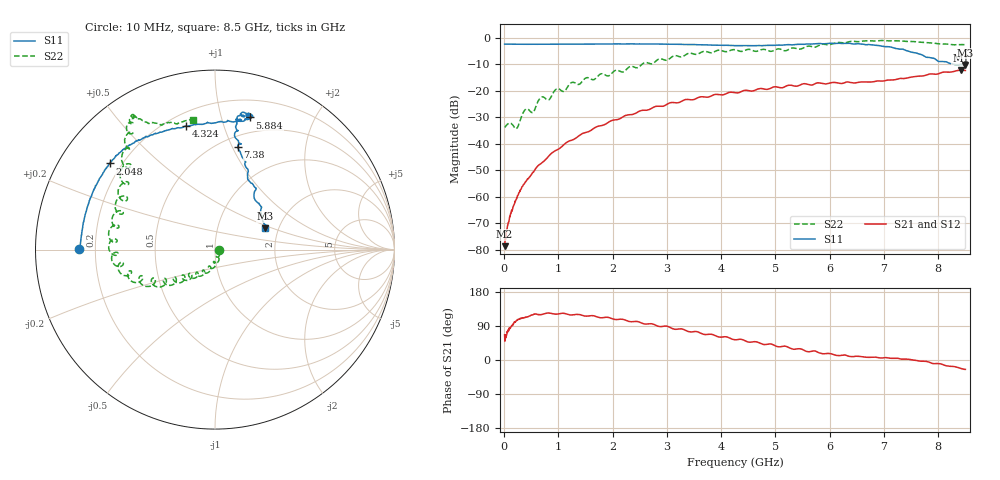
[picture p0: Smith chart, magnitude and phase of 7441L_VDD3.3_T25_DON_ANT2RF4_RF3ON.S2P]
!Agilent Technologies,E5071C,MY46417908,A.11.23
!Date: Mon May 03 19:54:31 2021
!Data & Calibration Information:
!Freq	S11:SOLT2(ON)	S21:SOLT2(ON)	S12:SOLT2(ON)	S22:SOLT2(ON)
!PortZ  Port1:50+j0  Port2:50+j0
!Above PortZ is port z conversion or system Z0 setting when saving the data.
!When reading, reference impedance value at option line is always used.
# Hz S dB R 50
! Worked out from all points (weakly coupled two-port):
!   1601 points, 10 MHz to 8.5 GHz, reference 50 ohm
!   highest |S21| = -12.28 dB at 8.415 GHz (marker M1); lowest = -78.7 dB at 10 MHz (marker M2)
!   lowest |S11| = -10.4 dB at 8.5 GHz (marker M3), VSWR 1.87, Z = 85.2 + j22.1 ohm
!   |S11| at or under -10 dB: 8.27 GHz to end of sweep
!   |S22| runs from -34.4 to -1.1 dB; largest |S21 - S12| = 0.0023
!   S11 on the Smith chart (normalised r, x): 10 MHz: 0.14, +0.00; 2.048 GHz: 0.16, +0.35; 4.324 GHz: 0.28, +0.76; 5.884 GHz: 0.35, +1.24; 7.38 GHz: 0.60, +1.05; 8.5 GHz: 1.70, +0.44
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1e7  -2.44 179.7  -78.70 66.1  -82.46 72.5  -33.87 -2.5
1.3735e8  -2.49 177.0  -65.28 89.9  -65.35 89.5  -32.53 -41.6
2.381688e8  -2.51 175.0  -60.48 104.8  -60.32 105.2  -34.15 -41.7
3.814375e8  -2.52 171.8  -54.81 112.2  -54.87 111.9  -27.39 -58.2
5.247062e8  -2.51 168.8  -51.07 119.1  -50.99 119.1  -28.30 -74.4
6.732812e8  -2.52 165.8  -47.63 119.6  -47.63 119.4  -22.66 -79.9
8.749188e8  -2.50 161.8  -43.68 122.6  -43.68 122.8  -22.06 -87.4
9.704312e8  -2.49 159.8  -42.45 121.1  -42.42 120.9  -19.36 -100.5
1.097781e9  -2.49 157.5  -40.47 123.4  -40.50 123.4  -20.35 -107.5
1.24105e9  -2.47 154.6  -38.77 118.7  -38.79 118.8  -17.01 -111.4
1.426769e9  -2.46 151.5  -36.39 118.5  -36.38 118.5  -16.88 -114.5
2.0476e9  -2.42 140.7  -31.05 106.8  -31.04 106.9  -12.42 -134.8
2.843538e9  -2.45 130.2  -25.91 88.9  -25.92 89.0  -8.19 -148.2
3.623556e9  -2.71 119.3  -22.36 70.8  -22.36 70.7  -5.64 -163.9
4.255e9  -3.04 104.7  -20.79 53.4  -20.79 53.4  -4.58 176.8
4.323981e9  -3.02 103.1  -20.79 54.5  -20.80 54.4  -5.03 173.9
5.671769e9  -2.44 75.1  -17.91 23.1  -17.86 23.1  -3.43 134.9
5.884019e9  -2.37 75.2  -17.41 16.4  -17.35 16.7  -2.51 131.6
7.088538e9  -3.44 79.5  -15.97 5.2  -16.01 5.2  -1.24 121.4
7.380381e9  -4.66 77.5  -15.44 2.3  -15.45 2.5  -1.39 120.7
8.4151e9  -10.10 26.5  -12.28 -22.3  -12.36 -22.2  -2.66 102.8
8.5e9  -10.37 22.8  -12.42 -24.7  -12.47 -24.7  -2.68 99.5
